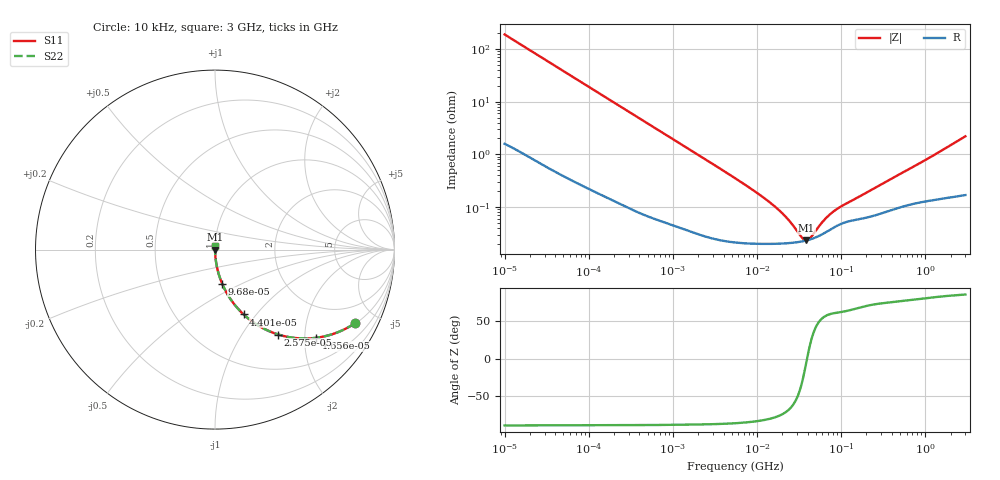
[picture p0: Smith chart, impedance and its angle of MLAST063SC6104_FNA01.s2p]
! MLAST063SC6104_FNA01  S-PARAMETER MODEL  ( Standard Model )
! Model Generated by TAIYO YUDEN Corporation (http://www.ty-top.com)
! Version 1.0
! TAIYO YUDEN Control No. 220601
! Copyright(c) 2014 TAIYO YUDEN CO.,LTD. All Rights Reserved.
! Product Description (link to TY-COMPAS)
! https://ds.yuden.co.jp/TYCOMPAS/or/detail?pn=MLAST063SC6104KFNA01&u=M
! Products Name : Multilayer Ceramic Capacitors
! Characteristics :
!  Capacitance : 0.1 [uF] , Rated Voltage : 25 [V] , TCC : X6S
!  Case Size : 0.6 x 0.3 / 0.024 x 0.012 [mm/inch] , Thickness : 0.3 / 0.012 [mm/inch]
!  (Conditions: Temperature = 25 [degC] , DC Bias Voltage = 0 [V])
! External Node Assignments :
!  1  o---| |---o  2
! GND o---------o GND
! Frequency Range : 10kHz  -  3GHz  [ 401 STEP ]
# MHZ S RI R 50
! Freq[MHz].  S11 Real  S11 Imag  S21 Real  S21 Imag  S12 Real  S12 Imag  S22 Real  S22 Imag
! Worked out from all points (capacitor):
!   401 points, 10 kHz to 3 GHz, reference 50 ohm
!   read as one part in series: C = 84.3 nF near 10.65 kHz
!   lowest |Z| = 23.3 mohm at 38.68 MHz (marker M1)
!   series resonance near 39.39 MHz, so ESL is about 190 pH
!   S11 on the Smith chart (normalised r, x): 10 kHz: 1.03, -3.77; 16.56 kHz: 1.02, -2.28; 25.75 kHz: 1.01, -1.47; 44.01 kHz: 1.01, -0.86; 96.8 kHz: 1.00, -0.39; 3 GHz: 1.00, +0.04
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0.01  0.7783 -0.4112  0.2217 0.4112  0.2217 0.4112  0.7783 -0.4112
0.012083  0.7075 -0.4506  0.2925 0.4506  0.2925 0.4506  0.7075 -0.4506
0.016561  0.5652 -0.4912  0.4348 0.4912  0.4348 0.4912  0.5652 -0.4912
0.02575  0.3527 -0.4732  0.6473 0.4732  0.6473 0.4732  0.3527 -0.4732
0.044011  0.1597 -0.3614  0.8403 0.3614  0.8403 0.3614  0.1597 -0.3614
0.058452  0.0984 -0.2927  0.9016 0.2927  0.9016 0.2927  0.0984 -0.2927
0.082683  0.0528 -0.2181  0.9472 0.2181  0.9472 0.2181  0.0528 -0.2181
0.096801  0.0395 -0.1891  0.9605 0.1891  0.9605 0.1891  0.0395 -0.1891
0.226771  0.00828 -0.084  0.9917 0.084  0.9917 0.084  0.00828 -0.084
0.683653  0.00136 -0.0283  0.9986 0.0283  0.9986 0.0283  0.00136 -0.0283
5.477226  0.000225 -0.00353  0.9998 0.00353  0.9998 0.00353  0.000225 -0.00353
10.61963  0.000203 -0.00172  0.9998 0.00172  0.9998 0.00172  0.000203 -0.00172
16.51234  0.000202 -0.000986  0.9998 0.000986  0.9998 0.000986  0.000202 -0.000986
23.35767  0.000206 -0.000549  0.9998 0.000549  0.9998 0.000549  0.000206 -0.000549
34.09912  0.000223 -0.000145  0.9998 0.000145  0.9998 0.000145  0.000223 -0.000145
38.68249  0.000233 -1.81e-05  0.9998 1.81e-05  0.9998 1.81e-05  0.000233 -1.81e-05
41.20027  0.000239 4.5e-05  0.9998 -4.5e-05  0.9998 -4.5e-05  0.000239 4.5e-05
45.28751  0.000251 0.00014  0.9997 -0.00014  0.9997 -0.00014  0.000251 0.00014
62.07353  0.000315 0.000456  0.9997 -0.000456  0.9997 -0.000456  0.000315 0.000456
85.08137  0.000424 0.000762  0.9996 -0.000762  0.9996 -0.000762  0.000424 0.000762
374.4521  0.000858 0.00317  0.9991 -0.00317  0.9991 -0.00317  0.000858 0.00317
3000  0.00216 0.0219  0.9978 -0.0219  0.9978 -0.0219  0.00216 0.0219
